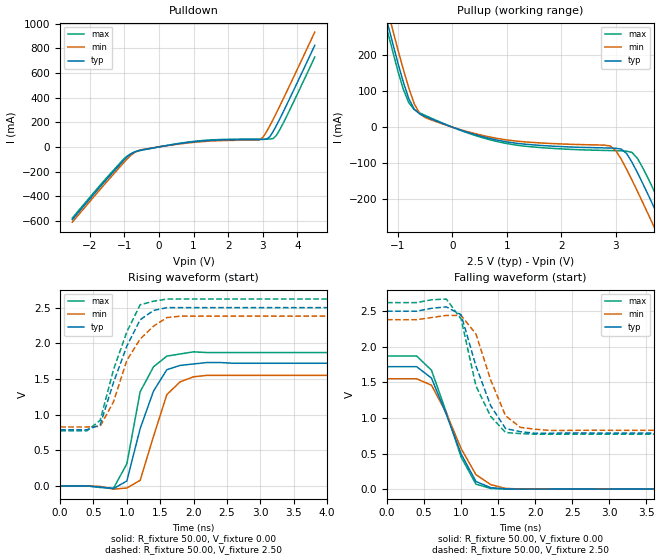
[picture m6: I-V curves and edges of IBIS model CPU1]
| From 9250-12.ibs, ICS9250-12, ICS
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|   Model CPU1
[Model]   CPU1
Model_type   Output
Polarity   Non-Inverting
Vmeas = 1.25V
Cref = 20pF
Rref = 0
Vref = 1.25V
C_comp   5.50pF   5.00pF   6.00pF
[Temperature Range]   27.00   70.00   0.00
[Voltage Range]   2.50V   2.38V   2.62V
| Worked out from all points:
|   slope of the pulldown table from 0 to 0.375 V, typ, clamps not added: 21.3 ohm
|   slope of the pullup table from 0 to 0.375 V, typ, clamps not added: 20 ohm
|   rising waveform, R_fixture 50.00, V_fixture 0.00: 20-80 % time 356ps typ, 311ps min, 288ps max; typ from 0 V to 1.72 V
|   rising waveform, R_fixture 50.00, V_fixture 2.50: 20-80 % time 414ps typ, 435ps min, 385ps max; typ from 0.787 V to 2.5 V
|   falling waveform, R_fixture 50.00, V_fixture 0.00: 20-80 % time 406ps typ, 429ps min, 381ps max; typ from 1.72 V to 0 V
|   falling waveform, R_fixture 50.00, V_fixture 2.50: 20-80 % time 344ps typ, 323ps min, 314ps max; typ from 2.5 V to 0.787 V
[Pulldown]
| voltage   I(typ)   I(min)   I(max)
-2.5V     -590.2mA   -611.1mA   -577.3mA
-1V       -103.4mA   -122.6mA   -93.34mA
-800mV    -56.35mA   -66.53mA   -54mA
-600mV    -31.06mA   -30.84mA   -33.09mA
1.2V      46.87mA    41.64mA    50.55mA
2.8V      59.89mA    54.8mA     63.4mA
3V        60.18mA    76.87mA    63.66mA
3.2V      81.83mA    169.7mA    63.99mA
3.3V      125.5mA    224.1mA    67.57mA
3.4V      177.7mA    280.3mA    96.49mA
3.7V      347.9mA    454.4mA    255.2mA
4.5V      824.4mA    932mA      729.3mA
[Pullup]
| voltage   I(typ)   I(min)   I(max)
-2.5V     1.06A      1.1A       1.04A
-1.6V     524.5mA    562.6mA    500.8mA
-1V       177.4mA    214.3mA    155.1mA
-800mV    78.91mA    108.5mA    67.55mA
-600mV    36.67mA    37.48mA    39.51mA
0V        268.7pA    568pA      1.46nA
2.9V      -57.91mA   -52.22mA   -64.86mA
3.3V      -97.17mA   -146.6mA   -70.06mA
3.7V      -220.5mA   -274.3mA   -174.4mA
3.9V      -285.6mA   -339.8mA   -238.8mA
4.1V      -351.5mA   -405.9mA   -304.4mA
4.5V      -484.6mA   -538.9mA   -437.2mA
[Ramp]
| variable   typ   min   max
dV/dt_r   1.03/255.90p   932.40m/270.64p   1.12/230.25p
dV/dt_f   1.03/200.00p   934.98m/200.00p   1.11/200.00p
[Rising Waveform]
R_fixture = 50.00
V_fixture = 0.00
V_fixture_min = 0.00
V_fixture_max = 0.00
| time   V(typ)   V(min)   V(max)
0s        0V         0V         0V
600ps     -16.26mV   -7mV       -22.09mV
800ps     -37.57mV   -45.67mV   -32.52mV
1ns       69.18mV    -29.49mV   309mV
1.2ns     804.3mV    78.14mV    1.32V
1.4ns     1.33V      694.9mV    1.67V
1.6ns     1.63V      1.28V      1.82V
1.8ns     1.69V      1.46V      1.85V
2.2ns     1.73V      1.55V      1.87V
10ns      1.72V      1.55V      1.87V
[Rising Waveform]
R_fixture = 50.00
V_fixture = 2.50
V_fixture_min = 2.38
V_fixture_max = 2.62
| time   V(typ)   V(min)   V(max)
0s        787.4mV    826.5mV    772.3mV
400ps     787.4mV    826.5mV    772.3mV
600ps     855.3mV    834.4mV    919.6mV
800ps     1.45V      1.18V      1.63V
1ns       1.96V      1.76V      2.16V
1.2ns     2.33V      2.06V      2.54V
1.4ns     2.46V      2.24V      2.59V
1.6ns     2.5V       2.36V      2.62V
1.8ns     2.5V       2.38V      2.62V
10ns      2.5V       2.38V      2.62V
[Falling Waveform]
R_fixture = 50.00
V_fixture = 0.00
V_fixture_min = 0.00
V_fixture_max = 0.00
| time   V(typ)   V(min)   V(max)
0s        1.72V      1.55V      1.87V
400ps     1.72V      1.55V      1.87V
600ps     1.56V      1.46V      1.67V
800ps     1.05V      1.07V      1.08V
1ns       495.1mV    569.7mV    450.3mV
1.2ns     107.3mV    203.5mV    70.12mV
1.4ns     20.37mV    63.29mV    9.46mV
1.6ns     4.12mV     10.42mV    1.22mV
1.8ns     -653uV     1.48mV     -28.55uV
10ns      5.57uV     -2.12uV    1.89uV
[Falling Waveform]
R_fixture = 50.00
V_fixture = 2.50
V_fixture_min = 2.38
V_fixture_max = 2.62
| time   V(typ)   V(min)   V(max)
0s        2.5V       2.38V      2.62V
400ps     2.5V       2.38V      2.62V
800ps     2.56V      2.44V      2.67V
1ns       2.45V      2.44V      2.39V
1.2ns     1.73V      2.18V      1.45V
1.4ns     1.17V      1.53V      1.02V
1.6ns     850.6mV    1.03V      795.5mV
1.8ns     806.5mV    867.3mV    779.6mV
2.2ns     785mV      824.4mV    770.6mV
10ns      787.4mV    826.5mV    772.3mV
